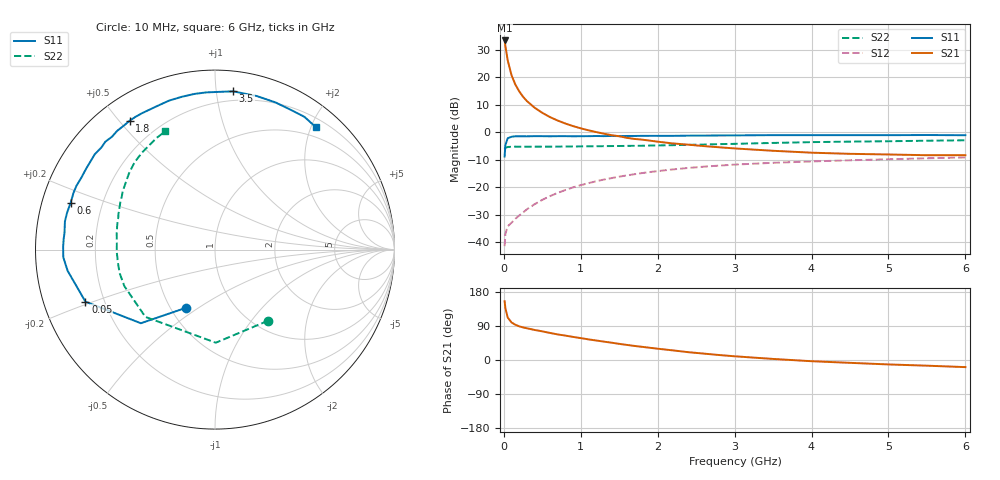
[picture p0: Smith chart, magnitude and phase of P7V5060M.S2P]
! SIEMENS Small Signal Semiconductors
! BFP196
! Si NPN RF Bipolar Junction Transistor in SOT143
! VCE = 0.5 V  IC = 60 mA
! Common Emitter S-Parameters:  May  1996
# GHz  S  MA  R  50
!  f  S11  S21  S12  S22
! GHz  MAG  ANG  MAG  ANG  MAG  ANG  MAG  ANG
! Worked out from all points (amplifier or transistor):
!   36 points, 10 MHz to 6 GHz, reference 50 ohm
!   highest |S21| = 33.5 dB at 10 MHz (marker M1)
!   |S21| within 3 dB of that: start of sweep to 25.94 MHz
!   unconditionally stable (mu >= 1): 217.3 MHz to end of sweep
!   at 250 MHz: K = 1.07, MAG = 19.5 dB, |S12| = -29.2 dB
!   at 1.4 GHz: K = 1.21, MAG = 5.1 dB, |S12| = -16.7 dB
!   at 6 GHz: K = 1.09, MAG = -1.4 dB, |S12| = -9.2 dB
!   S11 on the Smith chart (normalised r, x): 10 MHz: 0.60, -0.45; 50 MHz: 0.13, -0.19; 600 MHz: 0.09, +0.16; 1.8 GHz: 0.10, +0.53; 3.5 GHz: 0.13, +1.11; 6 GHz: 0.33, +2.08
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0.01  0.361 -116.3  47.19 155.0  0.0084 61.5  0.4942 -53.4
0.02  0.5822 -135.2  37.66 136.7  0.0141 49.9  0.5188 -89.5
0.05  0.7779 -158.1  20.55 112.3  0.0193 36.1  0.5395 -136.0
0.1  0.8295 -171.8  10.96 99.0  0.0225 38.3  0.5445 -158.1
0.15  0.8463 -177.1  7.395 93.0  0.0266 43.9  0.5472 -166.1
0.2  0.8462 179.0  5.571 88.8  0.0304 48.7  0.5455 -170.4
0.25  0.8452 176.1  4.436 86.0  0.0345 53.1  0.5462 -173.5
0.3  0.8437 173.7  3.706 83.7  0.0395 55.1  0.5455 -175.3
0.4  0.8509 169.3  2.805 79.3  0.0489 58.8  0.5474 -178.3
0.5  0.8495 166.0  2.262 75.6  0.0587 60.3  0.5473 179.4
0.6  0.8456 162.0  1.893 71.4  0.0686 61.2  0.5474 177.6
0.7  0.8495 158.1  1.636 67.5  0.0786 60.9  0.5482 176.0
0.8  0.8498 155.2  1.445 64.4  0.0887 60.3  0.5503 174.5
1.1  0.8497 144.9  1.087 54.4  0.1183 57.1  0.5557 170.4
1.4  0.857 135.4  0.886 45.7  0.1462 52.7  0.5609 166.5
1.8  0.8614 123.4  0.734 34.7  0.1808 46.1  0.5685 161.3
2.2  0.8618 112.7  0.626 25.3  0.2107 39.4  0.582 156.0
2.8  0.875 97.5  0.533 13.1  0.2472 29.6  0.6084 147.7
3.5  0.8875 83.5  0.46 2.8  0.278 19.0  0.6398 138.6
4.5  0.8865 67.7  0.405 -7.5  0.309 6.7  0.6759 127.1
5.5  0.8918 56.0  0.382 -15.0  0.336 -4.0  0.702 117.6
6  0.8835 50.5  0.383 -18.8  0.3484 -9.8  0.7149 112.9
